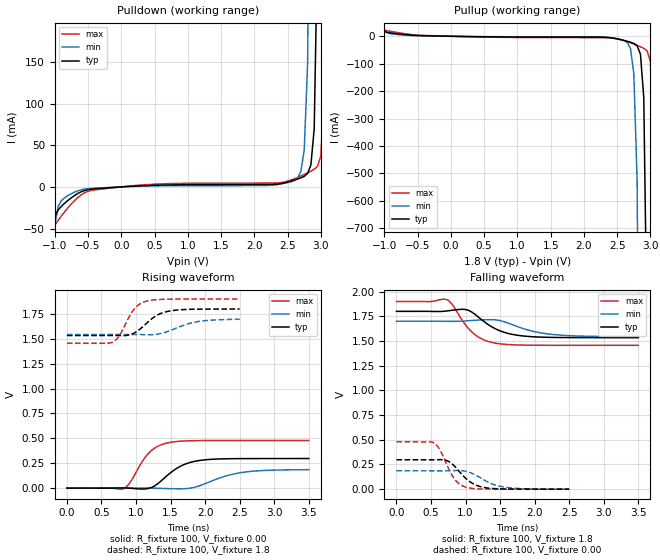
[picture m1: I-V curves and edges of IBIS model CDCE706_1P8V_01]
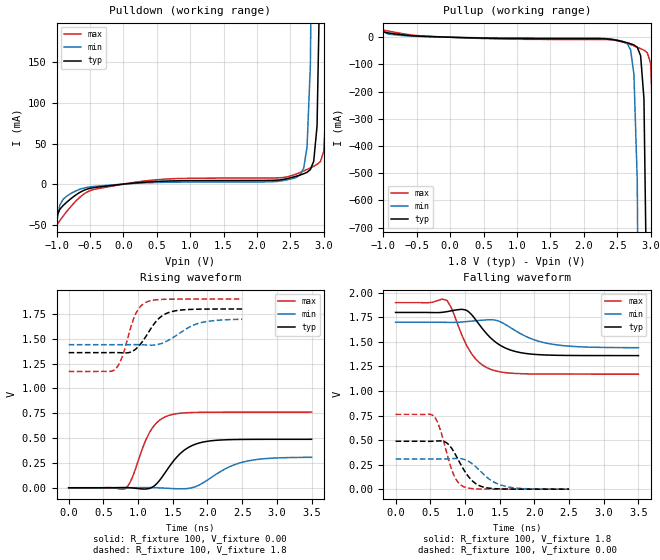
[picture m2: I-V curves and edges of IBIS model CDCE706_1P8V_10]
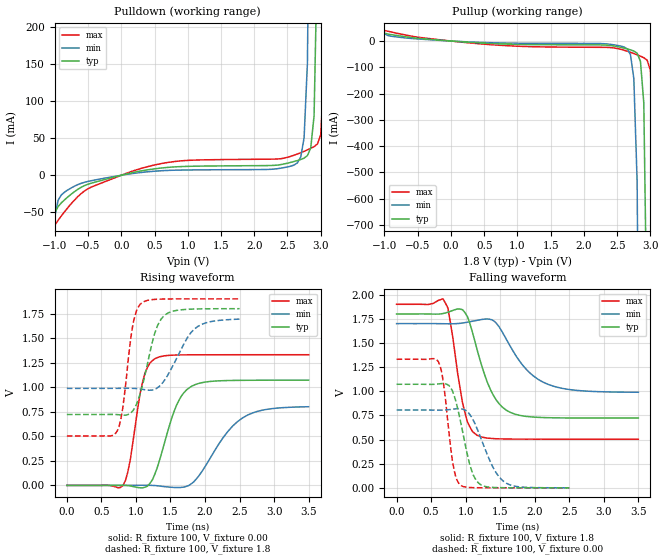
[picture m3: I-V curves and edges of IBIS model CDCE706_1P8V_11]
|   This file is an IBIS representation of the   |
|   Texas Instruments   |
|   CDCE706   |
|   PROGRAMMABLE 3-PLL CLOCK SYNTHESIZER / MULTIPLIER / DIVIDER   |
|   TSSOP20 Package   |
|=======================================================================mm===|
[IBIS Ver]   4.1
[File name]   scac072a.ibs
[File Rev]   1.00
[Date]   23th of Dec 2005
[Source]   file originated at Texas Instruments
|   this file was generated based on simulation results of TI-Spice
[Notes]  - The following information corresponds to the
|   CDCE706 input/output buffers and input ESD structures.
|   - No errors occured with the IBIS checker IBISCHK4 V4.1
|   The warnings can be ignored, as they have no impact to the
|   simulation results:
|   - Extreme currents - came from the extrapolation to -1.5V of
|   the INPUT GND/POWER_Clamp-Tables
|   - are normal, if a clamping diode is present
|   - The right simulation model should be selected by the model selector.
[Disclaimer]
  Texas Instruments Incorporated hereby grants the user of this IBIS
model a non-exclusive, nontransferable license to use this IBIS model
under the following terms.  Before using this IBIS model, the user
should read this license.  If the user does not accept these terms,
the IBIS model should be returned to Texas Instruments within 30 days.
  The user is granted this license only to use the IBIS model and
is not granted rights to sell, load, rent, lease or license the IBIS
model in whole or in part, or in modified form to anyone other than
user.  User may modify the IBIS model to suit its specific applications
but rights to derivative works and such modifications shall belong to
Texas Instruments.
  This IBIS model is provided on an "AS IS" basis and Texas Instruments
makes absolutely no warranty with respect to the information contained
herein.  TEXAS INSTRUMENTS DISCLAIMS AND CUSTOMER WAIVES ALL WARRANTIES,
EXPRESS OR IMPLIED, INCLUDING WARRANTIES OF MERCHANTABILITY OR FITNESS
FOR A PARTICULAR PURPOSE. The entire risk as to quality and performance
is with the Customer. ACCORDINGLY, IN NO EVENT SHALL THE COMPANY BE LIABLE
FOR ANY DAMAGES, WHETHER IN CONTRACT OR TORT,INCLUDING ANY LOST PROFITS
OR OTHER INCIDENTAL, CONSEQUENTIAL, EXEMPLARY, OR PUNITIVE DAMAGES ARISING
OUT OF THE USE OR APPLICATION OF THE IBIS model provided in this package.
Further, Texas Instruments reserves the right to discontinue or make changes
without notice to any product herein to improve reliability, function, or
design. Texas Instruments does not convey any license under patent rights
or any other intellectual property rights, including those of third parties.
Contact Texas Instruments at ATTN: HPA-High Speed Communication & Control, HSCC
IBIS Open Forum disclaims all warranties. See DISCLAIM.TXT
in vhdl.org:/pub/IBIS/models for the full disclaimer.
[Copyright]   Copyright (C) Texas Instruments Incorporated 2005
|   All rights reserved
|   Component   CDCE706
[Component]   CDCE706
[Manufacturer]   Texas Instruments Incorporated
[Package]
|   typ   min   max
R_pkg   50.07821m   41.7621m   59.7365m
L_pkg   2.8023nH   2.2481nH   3.5529nH
C_pkg   159.11fF   75.6975fF   279.7fF
[Pin] signal_name   model_name   R_pin   L_pin   C_pin
1   S0/A0/CLK_SEL sin0   5.54854E-02   3.46063E-09   2.75212E-13
2   S1/A1   sin0   5.51348E-02   3.14989E-09   1.89408E-13
3   VCC   POWER   4.21422E-02   2.61921E-09   1.60288E-13
4   GND   GND   4.48724E-02   2.27303E-09   7.56975E-14
5   CLK_IN0   clk_in0   4.47610E-02   2.24810E-09   8.40904E-14
6   CLK_IN1   clk_in1   4.49337E-02   2.27296E-09   8.52503E-14
7   VCC   POWER   4.44397E-02   2.32269E-09   7.93276E-14
8   GND   GND   4.63367E-02   2.70378E-09   1.65072E-13
9   SDATA   smbdatin   5.96533E-02   3.26534E-09   1.94459E-13
10   SCLOCK   smbclkin   5.72224E-02   3.50585E-09   2.75919E-13
11   Y0   cdce706_out   5.79869E-02   3.55290E-09   2.79700E-13
12   Y1   cdce706_out   5.80843E-02   3.19339E-09   1.90156E-13
13   GND   GND   4.17621E-02   2.70360E-09   1.65208E-13
14   VCCOUT1   POWER   4.61737E-02   2.39237E-09   8.15468E-14
15   Y2   cdce706_out   4.73305E-02   2.33399E-09   8.73366E-14
16   Y3   cdce706_out   4.68846E-02   2.29982E-09   8.55770E-14
17   GND   GND   4.74875E-02   2.34897E-09   7.80118E-14
18   VCCOUT2   POWER   4.52762E-02   2.67704E-09   1.60853E-13
19   Y4   cdce706_out   5.97365E-02   3.23519E-09   1.93061E-13
20   Y5   cdce706_out   5.58603E-02   3.48720E-09   2.76027E-13
[Pin Mapping] pulldown_ref pullup_ref gnd_clamp_ref power_clamp_ref ext_ref
1   GNDBUS   POWERBUSIN
2   GNDBUS   POWERBUSIN
3   NC   POWERBUSIN
4   GNDBUS   NC
5   GNDBUS   POWERBUSIN
6   GNDBUS   POWERBUSIN
7   NC   POWERBUSIN
8   GNDBUS   NC
9   GNDBUS   POWERBUSIN
10   GNDBUS   POWERBUSIN
11   GNDBUS   POWERBUSOUT1
12   GNDBUS   POWERBUSOUT1
13   GNDBUS   NC
14   NC   POWERBUSOUT1
15   GNDBUS   POWERBUSOUT2
16   GNDBUS   POWERBUSOUT2
17   GNDBUS   NC
18   NC   POWERBUSOUT2
19   GNDBUS   POWERBUSOUT2
20   GNDBUS   POWERBUSOUT2
[Diff Pin]  inv_pin  vdiff  tdelay_typ tdelay_min tdelay_max
5   6   200mV   NA   NA   NA
[Model Selector]   cdce706_out
CDCE706_3P3V_11   buffer with slew rate 3 @ 3.3V nom.
CDCE706_2P5V_11   buffer with slew rate 3 @ 2.5V nom.
CDCE706_1P8V_11   buffer with slew rate 3 @ 1.8V nom.
CDCE706_3P3V_10   buffer with slew rate 2 @ 3.3V nom.
CDCE706_3P3V_00   buffer with slew rate 0 @ 3.3V nom.
CDCE706_3P3V_01   buffer with slew rate 1 @ 3.3V nom.
CDCE706_2P5V_00   buffer with slew rate 0 @ 2.5V nom.
CDCE706_2P5V_01   buffer with slew rate 1 @ 2.5V nom.
CDCE706_2P5V_10   buffer with slew rate 2 @ 2.5V nom.
CDCE706_1P8V_10   buffer with slew rate 2 @ 1.8V nom.
CDCE706_1P8V_01   buffer with slew rate 1 @ 1.8V nom.
[Model Selector]   clk_in0
qlvcmos   input buffer with LVCMOS @ 3.3V nom.
qin   input buffer for quartz-crystal
qdiff   P input buffer for differential signal @ 3.3V nom.
[Model Selector]   clk_in1
qlvcmos   buffer with LVCMOS INPUT @ 3.3V nom.
qout   output buffer for quartz-crystal
qdiff   N input buffer for differential signal @ 3.3V nom.
| Models and submodels in the file (18): CDCE706_1P8V_01 (Output), CDCE706_1P8V_10 (Output), CDCE706_1P8V_11 (Output), CDCE706_2P5V_00 (Output), CDCE706_2P5V_01 (Output), CDCE706_2P5V_10 (Output), CDCE706_2P5V_11 (Output), CDCE706_3P3V_00 (Output), CDCE706_3P3V_01 (Output), CDCE706_3P3V_10 (Output), CDCE706_3P3V_11 (Output), sin0 (Input), qdiff (Input), qin (Input), qlvcmos (Input), qout (Output), smbclkin (Input), smbdatin (Input)
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|   Model   CDCE706_1P8V_01
[Model]   CDCE706_1P8V_01
Model_type   Output
Polarity   Non-Inverting
Vmeas  =   0.90V
Cref   =   3.00pF
Rref   =   60
Vref   =   0.90V
|Variable   typ   min   max
C_comp   1.503e-12   1.492e-12   1.525e-12
|Variable   typ   min   max
[Voltage range]   1.8   1.7   1.9
|Variable   typ   min   max
[Temperature range]  55   110   -15
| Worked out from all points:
|   slope of the pulldown table from 0 to 0.27 V, typ, clamps not added: 215 ohm
|   slope of the pullup table from 0 to 0.27 V, typ, clamps not added: 243 ohm
|   rising waveform, R_fixture 100, V_fixture 0.00: 20-80 % time 358ps typ, 482ps min, 283ps max; typ from 0 V to 0.297 V
|   falling waveform, R_fixture 100, V_fixture 1.8: 20-80 % time 387ps typ, 494ps min, 314ps max; typ from 1.8 V to 1.53 V
|   rising waveform, R_fixture 100, V_fixture 1.8: 20-80 % time 294ps typ, 384ps min, 218ps max; typ from 1.53 V to 1.8 V
|   falling waveform, R_fixture 100, V_fixture 0.00: 20-80 % time 267ps typ, 323ps min, 209ps max; typ from 0.298 V to 0 V
[Pulldown]
|Voltage   I(typ)   I(min)   I(max)
-1V       -36.37mA   -45.92mA   -46.21mA
-900mV    -23.24mA   -16.48mA   -34.83mA
-550mV    -4.261mA   -2.653mA   -6.929mA
2.55V     6.984mA    6.166mA    8.306mA
2.7V      10.89mA    18.66mA    13.11mA
2.75V     12.69mA    44.68mA    14.95mA
2.8V      16.07mA    146mA      16.9mA
2.85V     26.49mA    584.4mA    18.95mA
2.9V      69.95mA    2.552A     21.22mA
2.95V     295.1mA    2.552A     24.71mA
3V        1.576A     2.552A     37.26mA
3.1V      1.576A     2.552A     841.1mA
[Pullup]
|Voltage   I(typ)   I(min)   I(max)
-1V       17.31mA    19.45mA    22.5mA
2.25V     -3.226mA   -2.424mA   -5.045mA
2.65V     -18.21mA   -22.28mA   -19.5mA
2.7V      -21.77mA   -44.82mA   -23.75mA
2.75V     -26.21mA   -135.1mA   -28.33mA
2.8V      -34.7mA    -527.3mA   -33.23mA
2.85V     -65.56mA   -2.286A    -38.42mA
2.9V      -223.3mA   -2.286A    -44.19mA
2.95V     -1.114A    -2.286A    -53.35mA
3V        -1.114A    -2.286A    -92.33mA
3.05V     -1.114A    -2.286A    -406.7mA
3.1V      -1.114A    -2.286A    -3.303A
[Ramp]
|Variable   typ   min   max
dV/dt_r  9.014e-02/2.879e-10   5.605e-02/4.306e-10   0.1467/2.150e-10
dV/dt_f  8.047e-02/3.226e-10   4.722e-02/4.435e-10   0.1346/2.361e-10
R_load  =  50
[Rising Waveform]
R_fixture   =   100
V_fixture   =   0.00
V_fixture_min   =   0.00
V_fixture_max   =   0.00
C_fixture   =   0.00
|Time   V(typ)   V(min)   V(max)
0s        0V         0V         0V
813.1ps   1.932mV    8.249uV    -7.911mV
919.2ps   -903.5uV   371.5uV    61.36mV
1.096ns   -9.322mV   1.545mV    273.1mV
1.202ns   1.261mV    1.264mV    364.3mV
1.485ns   145.9mV    -5.338mV   458.6mV
1.697ns   237.3mV    -6.162mV   473.6mV
1.98ns    283.2mV    38.81mV    477.9mV
2.545ns   296.7mV    158.9mV    478.9mV
3.5ns     297.4mV    185.2mV    479mV
[Falling Waveform]
R_fixture   =   100
V_fixture   =   1.8
V_fixture_min   =   1.7
V_fixture_max   =   1.9
C_fixture   =   0.00
|Time   V(typ)   V(min)   V(max)
0s        1.8V       1.7V       1.9V
742.4ps   1.805V     1.699V     1.917V
813.1ps   1.812V     1.699V     1.866V
954.5ps   1.821V     1.701V     1.707V
1.096ns   1.79V      1.708V     1.587V
1.237ns   1.713V     1.713V     1.52V
1.449ns   1.618V     1.713V     1.476V
1.732ns   1.56V      1.65V      1.46V
2.227ns   1.537V     1.569V     1.456V
3.5ns     1.534V     1.544V     1.456V
[Rising Waveform]
R_fixture   =   100
V_fixture   =   1.8
V_fixture_min   =   1.7
V_fixture_max   =   1.9
C_fixture   =   0.00
|Time   V(typ)   V(min)   V(max)
0s        1.533V     1.543V     1.455V
656.6ps   1.534V     1.543V     1.465V
757.6ps   1.534V     1.543V     1.53V
959.6ps   1.553V     1.544V     1.787V
1.061ns   1.599V     1.543V     1.852V
1.162ns   1.662V     1.541V     1.88V
1.313ns   1.741V     1.548V     1.895V
1.515ns   1.783V     1.589V     1.899V
1.894ns   1.798V     1.673V     1.9V
2.5ns     1.8V       1.697V     1.9V
[Falling Waveform]
R_fixture   =   100
V_fixture   =   0.00
V_fixture_min   =   0.00
V_fixture_max   =   0.00
C_fixture   =   0.00
|Time   V(typ)   V(min)   V(max)
0s        297.7mV    186mV      479.4mV
555.6ps   297.8mV    185.5mV    463.7mV
606.1ps   298.9mV    185.3mV    425.1mV
707.1ps   294.3mV    185.7mV    282.5mV
833.3ps   237.7mV    188.1mV    109.9mV
909.1ps   179.1mV    188.3mV    52.96mV
1.01ns    104.7mV    180mV      19.04mV
1.212ns   26.29mV    116.4mV    2.76mV
1.54ns    2.451mV    23.94mV    470.9uV
2.5ns     196.1uV    381.2uV    253.1uV
|   Model   CDCE706_1P8V_10
[Model]   CDCE706_1P8V_10
Model_type   Output
Polarity   Non-Inverting
Vmeas  =   0.90V
Cref   =   3.00pF
Rref   =   60
Vref   =   0.90V
|Variable   typ   min   max
C_comp   1.524e-12   1.513e-12   1.546e-12
|Variable   typ   min   max
[Voltage range]   1.8   1.7   1.9
|Variable   typ   min   max
[Temperature range]  55   110   -15
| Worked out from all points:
|   slope of the pulldown table from 0 to 0.27 V, typ, clamps not added: 130 ohm
|   slope of the pullup table from 0 to 0.27 V, typ, clamps not added: 146 ohm
|   rising waveform, R_fixture 100, V_fixture 0.00: 20-80 % time 355ps typ, 481ps min, 270ps max; typ from 0 V to 0.488 V
|   falling waveform, R_fixture 100, V_fixture 1.8: 20-80 % time 383ps typ, 489ps min, 309ps max; typ from 1.8 V to 1.36 V
|   rising waveform, R_fixture 100, V_fixture 1.8: 20-80 % time 275ps typ, 372ps min, 197ps max; typ from 1.36 V to 1.8 V
|   falling waveform, R_fixture 100, V_fixture 0.00: 20-80 % time 257ps typ, 320ps min, 193ps max; typ from 0.488 V to 0 V
[Pulldown]
|Voltage   I(typ)   I(min)   I(max)
-1V       -39.53mA   -47.93mA   -50.91mA
-900mV    -26.27mA   -18.59mA   -39.26mA
-450mV    -4.44mA    -2.972mA   -6.803mA
2.4V      5.884mA    4.549mA    8.157mA
2.65V     11.32mA    11.73mA    14.46mA
2.75V     14.55mA    45.78mA    18.04mA
2.8V      17.93mA    147.1mA    19.99mA
2.85V     28.36mA    585.5mA    22.04mA
2.9V      71.82mA    2.553A     24.32mA
2.95V     297mA      2.553A     27.81mA
3V        1.578A     2.553A     40.37mA
3.1V      1.578A     2.553A     844.2mA
[Pullup]
|Voltage   I(typ)   I(min)   I(max)
-1V       19.97mA    21.05mA    26.4mA
2.25V     -5.283mA   -3.701mA   -8.4mA
2.65V     -20.3mA    -23.57mA   -22.9mA
2.7V      -23.86mA   -46.11mA   -27.15mA
2.75V     -28.3mA    -136.3mA   -31.74mA
2.8V      -36.8mA    -528.6mA   -36.64mA
2.85V     -67.65mA   -2.287A    -41.84mA
2.9V      -225.4mA   -2.287A    -47.62mA
2.95V     -1.116A    -2.287A    -56.77mA
3V        -1.116A    -2.287A    -95.77mA
3.05V     -1.116A    -2.287A    -410.1mA
3.1V      -1.116A    -2.287A    -3.307A
[Ramp]
|Variable   typ   min   max
dV/dt_r  0.1493/2.876e-10   9.311e-02/4.285e-10   0.2414/2.137e-10
dV/dt_f  0.1335/3.189e-10   7.848e-02/4.394e-10   0.2230/2.367e-10
R_load  =  50
[Rising Waveform]
R_fixture   =   100
V_fixture   =   0.00
V_fixture_min   =   0.00
V_fixture_max   =   0.00
C_fixture   =   0.00
|Time   V(typ)   V(min)   V(max)
0s        0V         0V         0V
813.1ps   1.808mV    8.09uV     -9.673mV
919.2ps   -1.964mV   382uV      107.7mV
1.167ns   -6.457mV   1.452mV    558.8mV
1.308ns   72.44mV    -1.424mV   679.2mV
1.449ns   212.6mV    -6.719mV   729.3mV
1.662ns   376.3mV    -10.02mV   753.4mV
1.944ns   461.2mV    53.01mV    759.9mV
2.545ns   486.6mV    264.5mV    761.1mV
3.5ns     487.7mV    306.4mV    761.3mV
[Falling Waveform]
R_fixture   =   100
V_fixture   =   1.8
V_fixture_min   =   1.7
V_fixture_max   =   1.9
C_fixture   =   0.00
|Time   V(typ)   V(min)   V(max)
0s        1.8V       1.7V       1.9V
742.4ps   1.808V     1.699V     1.921V
813.1ps   1.818V     1.699V     1.834V
954.5ps   1.832V     1.703V     1.57V
1.096ns   1.777V     1.712V     1.378V
1.237ns   1.647V     1.72V      1.271V
1.414ns   1.513V     1.724V     1.211V
1.732ns   1.401V     1.612V     1.178V
2.192ns   1.366V     1.485V     1.172V
3.5ns     1.361V     1.441V     1.172V
[Rising Waveform]
R_fixture   =   100
V_fixture   =   1.8
V_fixture_min   =   1.7
V_fixture_max   =   1.9
C_fixture   =   0.00
|Time   V(typ)   V(min)   V(max)
0s        1.36V      1.44V      1.171V
656.6ps   1.361V     1.44V      1.185V
757.6ps   1.359V     1.44V      1.292V
959.6ps   1.392V     1.441V     1.743V
1.035ns   1.447V     1.44V      1.826V
1.111ns   1.521V     1.438V     1.866V
1.288ns   1.696V     1.442V     1.894V
1.465ns   1.77V      1.495V     1.899V
1.894ns   1.798V     1.66V      1.9V
2.5ns     1.8V       1.696V     1.9V
[Falling Waveform]
R_fixture   =   100
V_fixture   =   0.00
V_fixture_min   =   0.00
V_fixture_max   =   0.00
C_fixture   =   0.00
|Time   V(typ)   V(min)   V(max)
0s        488.1mV    307.7mV    761.9mV
555.6ps   488.9mV    306.9mV    741.6mV
631.3ps   491.7mV    306.7mV    632.8mV
732.3ps   472.9mV    308.3mV    383.4mV
833.3ps   388.5mV    312.2mV    154.8mV
909.1ps   291.6mV    312.5mV    62.51mV
984.8ps   196.5mV    304.5mV    24.64mV
1.212ns   34.49mV    190.7mV    2.004mV
1.54ns    2.42mV     37.16mV    499.8uV
2.5ns     255uV      483.8uV    295.9uV
|   Model   CDCE706_1P8V_11
[Model]   CDCE706_1P8V_11
Model_type   Output
Polarity   Non-Inverting
Vmeas  =   0.90V
Cref   =   3.00pF
Rref   =   60
Vref   =   0.90V
|Variable   typ   min   max
C_comp   1.546e-12   1.541e-12   1.551e-12
|Variable   typ   min   max
[Voltage range]   1.8   1.7   1.9
|Variable   typ   min   max
[Temperature range]  55   110   -15
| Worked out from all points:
|   slope of the pulldown table from 0 to 0.27 V, typ, clamps not added: 50.4 ohm
|   slope of the pullup table from 0 to 0.27 V, typ, clamps not added: 56.6 ohm
|   rising waveform, R_fixture 100, V_fixture 0.00: 20-80 % time 293ps typ, 485ps min, 181ps max; typ from 0 V to 1.07 V
|   falling waveform, R_fixture 100, V_fixture 1.8: 20-80 % time 310ps typ, 459ps min, 189ps max; typ from 1.8 V to 0.723 V
|   rising waveform, R_fixture 100, V_fixture 1.8: 20-80 % time 227ps typ, 327ps min, 144ps max; typ from 0.722 V to 1.8 V
|   falling waveform, R_fixture 100, V_fixture 0.00: 20-80 % time 199ps typ, 290ps min, 129ps max; typ from 1.07 V to 0 V
[Pulldown]
|Voltage   I(typ)   I(min)   I(max)
-1V       -51.15mA   -55.9mA    -67.5mA
-700mV    -21.94mA   -14.61mA   -33.21mA
300mV     5.856mA    3.768mA    9.275mA
2.5V      16.3mA     11.26mA    24.3mA
2.65V     19.93mA    16.81mA    28.76mA
2.75V     23.19mA    50.87mA    32.38mA
2.8V      26.59mA    152.2mA    34.35mA
2.85V     37.02mA    590.6mA    36.42mA
2.9V      80.5mA     2.558A     38.71mA
2.95V     305.7mA    2.558A     42.23mA
3V        1.587A     2.558A     54.8mA
3.1V      1.587A     2.558A     858.7mA
[Pullup]
|Voltage   I(typ)   I(min)   I(max)
-1V       30.07mA    28.02mA    40.27mA
400mV     -6.753mA   -4.753mA   -9.897mA
2.25V     -14.83mA   -9.641mA   -23.94mA
2.65V     -29.98mA   -29.58mA   -38.67mA
2.7V      -33.55mA   -52.13mA   -42.95mA
2.75V     -38.01mA   -142.4mA   -47.56mA
2.8V      -46.52mA   -534.7mA   -52.48mA
2.85V     -77.39mA   -2.294A    -57.71mA
2.9V      -235.2mA   -2.294A    -63.51mA
2.95V     -1.126A    -2.294A    -72.69mA
3V        -1.126A    -2.294A    -111.7mA
3.05V     -1.126A    -2.294A    -426.1mA
[Ramp]
|Variable   typ   min   max
dV/dt_r  0.4016/3.140e-10   0.2607/4.749e-10   0.5731/2.029e-10
dV/dt_f  0.3703/2.979e-10   0.2210/4.105e-10   0.5881/2.123e-10
R_load  =  50
[Rising Waveform]
R_fixture   =   100
V_fixture   =   0.00
V_fixture_min   =   0.00
V_fixture_max   =   0.00
C_fixture   =   0.00
|Time   V(typ)   V(min)   V(max)
0s        0V         0V         0V
813.1ps   1.821mV    10.22uV    -74.46uV
919.2ps   -5.65mV    468.6uV    265.6mV
1.096ns   -24.8mV    1.981mV    1.052V
1.273ns   112.8mV    -1.185mV   1.29V
1.591ns   821.9mV    -21.48mV   1.328V
1.803ns   1.009V     17.69mV    1.33V
2.333ns   1.068V     551.9mV    1.331V
2.545ns   1.07V      688mV      1.331V
3.5ns     1.072V     801.2mV    1.331V
[Falling Waveform]
R_fixture   =   100
V_fixture   =   1.8
V_fixture_min   =   1.7
V_fixture_max   =   1.9
C_fixture   =   0.00
|Time   V(typ)   V(min)   V(max)
0s        1.8V       1.7V       1.9V
671.7ps   1.804V     1.699V     1.956V
742.4ps   1.818V     1.698V     1.863V
989.9ps   1.814V     1.71V      778.9mV
1.167ns   1.428V     1.734V     543.4mV
1.379ns   987.8mV    1.74V      511.3mV
1.662ns   776.8mV    1.445V     505.3mV
1.909ns   737.2mV    1.204V     504.3mV
2.227ns   726mV      1.063V     504.2mV
3.5ns     722.7mV    989.7mV    504mV
[Rising Waveform]
R_fixture   =   100
V_fixture   =   1.8
V_fixture_min   =   1.7
V_fixture_max   =   1.9
C_fixture   =   0.00
|Time   V(typ)   V(min)   V(max)
0s        722.1mV    988.1mV    503.6mV
732.3ps   720.8mV    988.6mV    558.5mV
808.1ps   715.4mV    989.1mV    780.9mV
909.1ps   729.4mV    989.2mV    1.41V
959.6ps   763.2mV    988.3mV    1.653V
1.086ns   997.5mV    979.7mV    1.858V
1.263ns   1.528V     977.1mV    1.894V
1.414ns   1.732V     1.072V     1.898V
1.843ns   1.796V     1.591V     1.899V
2.5ns     1.8V       1.693V     1.9V
[Falling Waveform]
R_fixture   =   100
V_fixture   =   0.00
V_fixture_min   =   0.00
V_fixture_max   =   0.00
C_fixture   =   0.00
|Time   V(typ)   V(min)   V(max)
0s        1.072V     806.1mV    1.331V
606.1ps   1.076V     804.3mV    1.305V
681.8ps   1.079V     805.3mV    1.066V
808.1ps   1.006V     813.7mV    279.8mV
909.1ps   743.5mV    819.5mV    37.32mV
1.061ns   238.1mV    758.3mV    3.672mV
1.212ns   35.07mV    529mV      1.18mV
1.414ns   4.077mV    189.6mV    552.4uV
1.591ns   1.405mV    47.41mV    410uV
2.5ns     309.7uV    579.3uV    296.8uV
